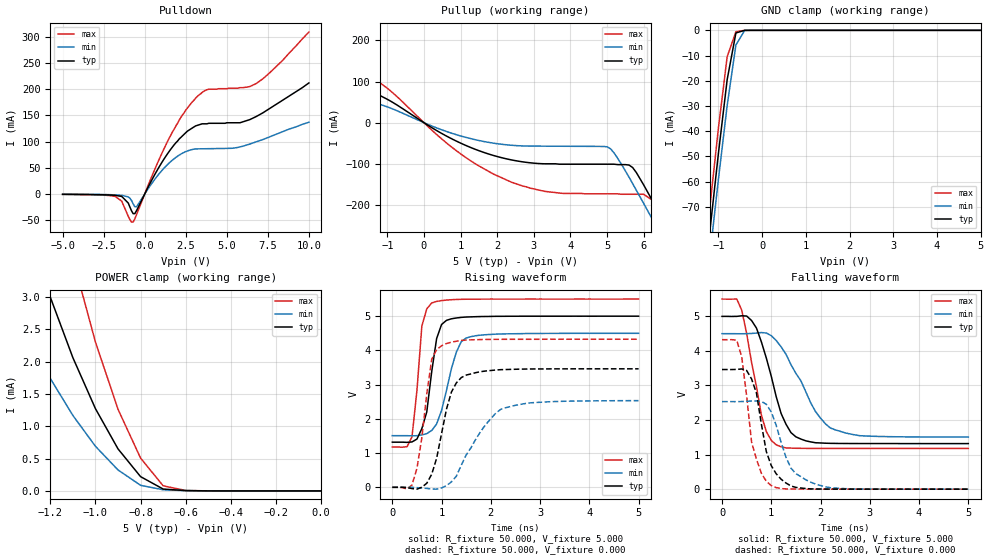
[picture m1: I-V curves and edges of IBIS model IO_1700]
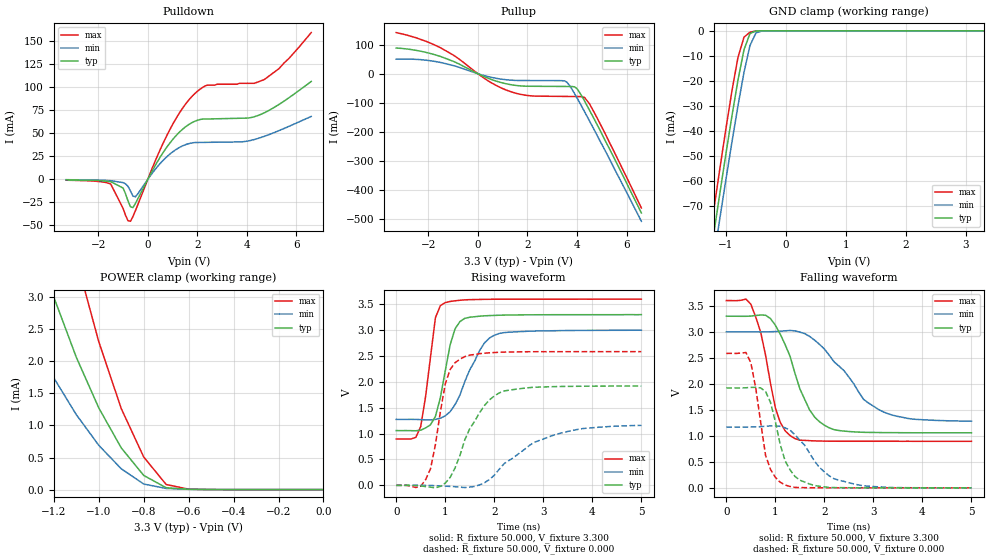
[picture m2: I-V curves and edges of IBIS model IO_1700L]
| / 7\'7   Xilinx XC1700 I/O Buffer IBIS File
| \ \   Xilinx Inc.
| / /   2100 Logic Drive
| \_\/.\   San Jose,   CA 95124
[IBIS ver]   2.1
[File name]   xc1700.ibs
[File Rev]   1.0
[Date]   July 26, 1999
[Source]   Spice netlist
[Notes]   - Best/worse process data included in the model
   - Created by Joey Jia x4437
[Disclaimer] The data in this model is derived from SPICE simulations
   using modeling information extracted from the target pro-
   cess. While a great deal of care has been take to provide
   information that is accurate, this model is considered
   preliminary as it has not been verified by actual silicon
   measurement. Treat the data in this model as preliminary
   until actual silicon verification is performed.
[Copyright]   Xilinx Inc. All right reserved
|   Component XC1701_PC20
[Component]   XC1701_PC20
[Manufacturer]   Xilinx Inc.
[Package]
| variable   typ   min   max
R_pkg   53.00m   49.000m   57.00m
L_pkg   3.125nH   2.880nH   3.370nH
C_pkg   0.650pF   0.630pF   0.670pF
[Pin]  signal_name   model_name   R_pin   L_pin   C_pin
io   datap   IO_1700   NA   NA   NA
| End [Component] XC1701_PC20
|   Component XC1701_PD8
[Component]   XC1701_PD8
[Manufacturer]   Xilinx Inc.
[Package]
| variable   typ   min   max
R_pkg   89.00m   80.000m   98.00m
L_pkg   5.840nH   4.160nH   7.520nH
C_pkg   0.935pF   0.720pF   1.150pF
[Pin]  signal_name   model_name   R_pin   L_pin   C_pin
io   datap   IO_1700   NA   NA   NA
| End [Component] XC1701_PD8
|   Component XC1701_SO20
[Component]   XC1701_SO20
[Manufacturer]   Xilinx Inc.
[Package]
| variable   typ   min   max
R_pkg   51.50m   44.000m   59.00m
L_pkg   3.155nH   1.960nH   4.350nH
C_pkg   0.585pF   0.350pF   0.820pF
[Pin]  signal_name   model_name   R_pin   L_pin   C_pin
io   datap   IO_1700   NA   NA   NA
| End [Component] XC1701_SO20
|   Component XC1701L_PC20
[Component]   XC1701L_PC20
[Manufacturer]   Xilinx Inc.
[Package]
| variable   typ   min   max
R_pkg   53.00m   49.000m   57.00m
L_pkg   3.125nH   2.880nH   3.370nH
C_pkg   0.650pF   0.630pF   0.670pF
[Pin]  signal_name   model_name   R_pin   L_pin   C_pin
io   datap   IO_1700L   NA   NA   NA
| End [Component] XC1701L_PC20
|   Component XC1701L_PD8
[Component]   XC1701L_PD8
[Manufacturer]   Xilinx Inc.
[Package]
| variable   typ   min   max
R_pkg   89.00m   80.000m   98.00m
L_pkg   5.840nH   4.160nH   7.520nH
C_pkg   0.935pF   0.720pF   1.150pF
[Pin]  signal_name   model_name   R_pin   L_pin   C_pin
io   datap   IO_1700L   NA   NA   NA
| End [Component] XC1701L_PD8
|   Component XC1701L_SO20
[Component]   XC1701L_SO20
[Manufacturer]   Xilinx Inc.
[Package]
| variable   typ   min   max
R_pkg   51.50m   44.000m   59.00m
L_pkg   3.155nH   1.960nH   4.350nH
C_pkg   0.585pF   0.350pF   0.820pF
[Pin]  signal_name   model_name   R_pin   L_pin   C_pin
io   datap   IO_1700L   NA   NA   NA
| End [Component] XC1701L_SO20
|   Component XC1702_PC44
[Component]   XC1702_PC44
[Manufacturer]   Xilinx Inc.
[Package]
| variable   typ   min   max
R_pkg   67.50m   66.000m   69.00m
L_pkg   3.905nH   3.550nH   4.260nH
C_pkg   0.895pF   0.790pF   1.000pF
[Pin]  signal_name   model_name   R_pin   L_pin   C_pin
io   datap   IO_1700L   NA   NA   NA
| End [Component] XC1702_PC44
|   Component XC1702_VQ44
[Component]   XC1702_VQ44
[Manufacturer]   Xilinx Inc.
[Package]
| variable   typ   min   max
R_pkg   54.15m   51.300m   57.00m
L_pkg   2.157nH   1.995nH   2.309nH
C_pkg   0.261pF   0.247pF   0.276pF
[Pin]  signal_name   model_name   R_pin   L_pin   C_pin
io   datap   IO_1700L   NA   NA   NA
| End [Component] XC1702_VQ44
|   Component XC1704_PC44
[Component]   XC1704_PC44
[Manufacturer]   Xilinx Inc.
[Package]
| variable   typ   min   max
R_pkg   67.50m   66.000m   69.00m
L_pkg   3.905nH   3.550nH   4.260nH
C_pkg   0.895pF   0.790pF   1.000pF
[Pin]  signal_name   model_name   R_pin   L_pin   C_pin
io   datap   IO_1700L   NA   NA   NA
| End [Component] XC1704_PC44
|   Component XC1704_VQ44
[Component]   XC1704_VQ44
[Manufacturer]   Xilinx Inc.
[Package]
| variable   typ   min   max
R_pkg   54.15m   51.300m   57.00m
L_pkg   2.157nH   1.995nH   2.309nH
C_pkg   0.261pF   0.247pF   0.276pF
[Pin]  signal_name   model_name   R_pin   L_pin   C_pin
io   datap   IO_1700L   NA   NA   NA
| End [Component] XC1704_VQ44
|   Component XC17512_PC20
[Component]   XC17512_PC20
[Manufacturer]   Xilinx Inc.
[Package]
| variable   typ   min   max
R_pkg   53.00m   49.000m   57.00m
L_pkg   3.125nH   2.880nH   3.370nH
C_pkg   0.650pF   0.630pF   0.670pF
[Pin]  signal_name   model_name   R_pin   L_pin   C_pin
io   datap   IO_1700   NA   NA   NA
| End [Component] XC17512_PC20
|   Component XC17512_PD8
[Component]   XC17512_PD8
[Manufacturer]   Xilinx Inc.
[Package]
| variable   typ   min   max
R_pkg   89.00m   80.000m   98.00m
L_pkg   5.840nH   4.160nH   7.520nH
C_pkg   0.935pF   0.720pF   1.150pF
[Pin]  signal_name   model_name   R_pin   L_pin   C_pin
io   datap   IO_1700   NA   NA   NA
| End [Component] XC17512_PD8
|   Component XC17512_SO20
[Component]   XC17512_SO20
[Manufacturer]   Xilinx Inc.
[Package]
| variable   typ   min   max
R_pkg   51.50m   44.000m   59.00m
L_pkg   3.155nH   1.960nH   4.350nH
C_pkg   0.585pF   0.350pF   0.820pF
[Pin]  signal_name   model_name   R_pin   L_pin   C_pin
io   datap   IO_1700   NA   NA   NA
| End [Component] XC17512_SO20
|   Component XC17512L_PC20
[Component]   XC17512L_PC20
[Manufacturer]   Xilinx Inc.
[Package]
| variable   typ   min   max
R_pkg   53.00m   49.000m   57.00m
L_pkg   3.125nH   2.880nH   3.370nH
C_pkg   0.650pF   0.630pF   0.670pF
[Pin]  signal_name   model_name   R_pin   L_pin   C_pin
io   datap   IO_1700L   NA   NA   NA
| End [Component] XC17512L_PC20
|   Component XC17512L_PD8
[Component]   XC17512L_PD8
[Manufacturer]   Xilinx Inc.
[Package]
| variable   typ   min   max
R_pkg   89.00m   80.000m   98.00m
L_pkg   5.840nH   4.160nH   7.520nH
C_pkg   0.935pF   0.720pF   1.150pF
[Pin]  signal_name   model_name   R_pin   L_pin   C_pin
io   datap   IO_1700L   NA   NA   NA
| End [Component] XC17512L_PD8
|   Component XC17512L_SO20
[Component]   XC17512L_SO20
[Manufacturer]   Xilinx Inc.
[Package]
| variable   typ   min   max
R_pkg   51.50m   44.000m   59.00m
L_pkg   3.155nH   1.960nH   4.350nH
C_pkg   0.585pF   0.350pF   0.820pF
[Pin]  signal_name   model_name   R_pin   L_pin   C_pin
io   datap   IO_1700L   NA   NA   NA
| End [Component] XC17512L_SO20
| Models and submodels in the file (2): IO_1700 (I/O), IO_1700L (I/O)
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|   Model IO_1700
[Model]   IO_1700
Model_type   I/O
Polarity   Non-Inverting
Enable   Active-High
Vinl =   0.800V
Vinh =   2.000V
Vmeas =   2.500V
Cref =  50.000pF
Rref =   1.000M
Vref =  0.000V
C_comp   2.750pF   2.250pF   3.250pF
[Temperature Range]   50.000   100.000   0.000
[Voltage Range]   5.000V   4.500V   5.500V
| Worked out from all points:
|   slope of the pulldown table from 0 to 0.75 V, typ, clamps not added: 16.8 ohm
|   slope of the pullup table from 0 to 0.75 V, typ, clamps not added: 19.3 ohm
|   GND clamp passes 1 mA (typ) near -0.59 V on its own axis
|   POWER clamp passes 1 mA (typ) near -0.96 V on its own axis
|   rising waveform, R_fixture 50.000, V_fixture 5.000: 20-80 % time 222ps typ, 325ps min, 154ps max; typ from 1.32 V to 5 V
|   rising waveform, R_fixture 50.000, V_fixture 0.000: 20-80 % time 331ps typ, 657ps min, 237ps max; typ from 0 V to 3.46 V
|   falling waveform, R_fixture 50.000, V_fixture 5.000: 20-80 % time 444ps typ, 672ps min, 339ps max; typ from 5 V to 1.32 V
|   falling waveform, R_fixture 50.000, V_fixture 0.000: 20-80 % time 296ps typ, 409ps min, 267ps max; typ from 3.46 V to 0 V
[Pulldown]
| voltage   I(typ)   I(min)   I(max)
-5V       -500uA     -400uA     -700uA
-1.8V     -2.5mA     -1.6mA     -4.5mA
-1.4V     -4.5mA     -2.4mA     -13.5mA
-1V       -17.19mA   -5.5mA     -42.5mA
-700mV    -37.46mA   -18.93mA   -53.28mA
-500mV    -31.8mA    -24.06mA   -39.58mA
1.4V      77.3mA     56.57mA    101mA
3.1V      130mA      86.12mA    183mA
3.9V      135mA      86.54mA    200mA
5.8V      136mA      89.89mA    203mA
6.8V      148mA      99.73mA    211mA
10V       212mA      137mA      309mA
[Pullup]
| voltage   I(typ)   I(min)   I(max)
-5V       138mA      75.48mA    233mA
-3.8V     136mA      79.24mA    211mA
-2.2V     104mA      68.39mA    154mA
-1V       56.81mA    38.43mA    83.6mA
1V        -49.62mA   -32.24mA   -75.63mA
2.4V      -90.7mA    -55.01mA   -145mA
3.3V      -100mA     -57.13mA   -167mA
5V        -101mA     -58.64mA   -173mA
5.7V      -109mA     -148mA     -174mA
6.4V      -215mA     -261mA     -198mA
6.8V      -281mA     -327mA     -262mA
10V       -833mA     -863mA     -828mA
[GND_clamp]
| voltage   I(typ)   I(min)   I(max)
-5V       -728mA     -719mA     -739mA
-1.4V     -113mA     -121mA     -104mA
-1.2V     -80.19mA   -89.89mA   -70.7mA
-1V       -48.75mA   -59.03mA   -38.71mA
-800mV    -19.55mA   -29.76mA   -10.47mA
-600mV    -1.037mA   -5.805mA   -545uA
-400mV    -3.699uA   -72.4uA    -2.038uA
5V        350pA      999nA      143pA
[POWER_clamp]
| voltage   I(typ)   I(min)   I(max)
-5V       71.66mA    42.52mA    116mA
-1.4V     5.246mA    3.126mA    8.7mA
-1.3V     4.067mA    2.398mA    6.818mA
-1.2V     3.001mA    1.742mA    5.11mA
-1.1V     2.064mA    1.169mA    3.598mA
-1V       1.274mA    691uA      2.306mA
-900mV    651uA      325uA      1.264mA
-800mV    221uA      87.03uA    508uA
-700mV    28.94uA    18.03uA    79.19uA
-600mV    5.041uA    4.416uA    6.917uA
0V        350pA      2.497nA    186pA
[Ramp]
| variable   typ   min   max
dV/dt_r   2.077/0.321n   1.520/0.637n   2.596/0.184n
dV/dt_f   2.209/0.440n   1.795/0.668n   2.593/0.308n
R_load = 50.000
[Rising Waveform]
R_fixture = 50.000
V_fixture = 5.000
V_fixture_min = 4.500
V_fixture_max = 5.500
L_fixture = 0.000H
C_fixture = 0.000F
| time   V(typ)   V(min)   V(max)
0s        1.319V     1.509V     1.178V
400ps     1.326V     1.504V     1.474V
600ps     1.716V     1.53V      4.712V
700ps     2.203V     1.569V     5.214V
800ps     3.381V     1.66V      5.387V
900ps     4.347V     1.851V     5.431V
1ns       4.757V     2.245V     5.455V
1.3ns     4.947V     3.95V      5.488V
1.5ns     4.975V     4.362V     5.495V
5ns       5V         4.499V     5.5V
[Rising Waveform]
R_fixture = 50.000
V_fixture = 0.000
V_fixture_min = 0.000
V_fixture_max = 0.000
L_fixture = 0.000H
C_fixture = 0.000F
| time   V(typ)   V(min)   V(max)
0s        0V         0V         0V
400ps     -36.91mV   -1.493mV   68.88mV
600ps     2.791mV    -20.69mV   1.452V
800ps     381mV      -52.4mV    3.743V
1ns       1.57V      -19.69mV   4.136V
1.2ns     2.782V     158mV      4.242V
1.3ns     3.05V      324mV      4.268V
1.8ns     3.38V      1.644V     4.317V
2.2ns     3.437V     2.277V     4.324V
5ns       3.462V     2.533V     4.326V
[Falling Waveform]
R_fixture = 50.000
V_fixture = 5.000
V_fixture_min = 4.500
V_fixture_max = 5.500
L_fixture = 0.000H
C_fixture = 0.000F
| time   V(typ)   V(min)   V(max)
0s        5V         4.5V       5.5V
300ps     5V         4.498V     5.501V
400ps     5.017V     4.497V     5.182V
600ps     4.881V     4.506V     3.67V
800ps     4.259V     4.532V     2.14V
1.1ns     2.678V     4.303V     1.284V
1.4ns     1.636V     3.604V     1.189V
1.9ns     1.343V     2.242V     1.179V
2.2ns     1.326V     1.77V      1.179V
5ns       1.319V     1.509V     1.178V
[Falling Waveform]
R_fixture = 50.000
V_fixture = 0.000
V_fixture_min = 0.000
V_fixture_max = 0.000
L_fixture = 0.000H
C_fixture = 0.000F
| time   V(typ)   V(min)   V(max)
0s        3.462V     2.534V     4.326V
300ps     3.466V     2.533V     4.308V
400ps     3.478V     2.535V     3.832V
600ps     3.19V      2.551V     1.364V
700ps     2.777V     2.552V     865mV
800ps     1.875V     2.538V     458mV
1ns       681mV      2.234V     103mV
1.4ns     92.11mV    608mV      4.998mV
1.8ns     7.997mV    202mV      1.287mV
5ns       186uV      382uV      121uV
|   Model IO_1700L
[Model]   IO_1700L
Model_type   I/O
Polarity   Non-Inverting
Enable   Active-High
Vinl =   0.800V
Vinh =   2.000V
Vmeas =   1.650V
Cref =  50.000pF
Rref =   1.000M
Vref =  0.000V
C_comp   2.750pF   2.250pF   3.250pF
[Temperature Range]   50.000   100.000   0.000
[Voltage Range]   3.300V   3.000V   3.600V
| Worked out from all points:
|   slope of the pulldown table from 0 to 0.495 V, typ, clamps not added: 20.8 ohm
|   slope of the pullup table from 0 to 0.495 V, typ, clamps not added: 27 ohm
|   GND clamp passes 1 mA (typ) near -0.60 V on its own axis
|   POWER clamp passes 1 mA (typ) near -0.96 V on its own axis
|   rising waveform, R_fixture 50.000, V_fixture 3.300: 20-80 % time 295ps typ, 502ps min, 225ps max; typ from 1.06 V to 3.3 V
|   rising waveform, R_fixture 50.000, V_fixture 0.000: 20-80 % time 575ps typ, 1.05ns min, 297ps max; typ from 0 V to 1.92 V
|   falling waveform, R_fixture 50.000, V_fixture 3.300: 20-80 % time 543ps typ, 897ps min, 359ps max; typ from 3.3 V to 1.06 V
|   falling waveform, R_fixture 50.000, V_fixture 0.000: 20-80 % time 348ps typ, 613ps min, 271ps max; typ from 1.92 V to 0 V
[Pulldown]
| voltage   I(typ)   I(min)   I(max)
-3.3V     -600uA     -400uA     -1mA
-1.5V     -2.5mA     -1.5mA     -5mA
-1V       -9.44mA    -3.56mA    -31.42mA
-800mV    -23.41mA   -7.59mA    -44.81mA
-700mV    -29.72mA   -12.65mA   -45.51mA
-500mV    -26.19mA   -18.96mA   -34.02mA
700mV     32.2mA     22.71mA    43.69mA
1.8V      61.63mA    39.51mA    90.28mA
2.4V      65.36mA    40.06mA    102mA
4.7V      71.97mA    46.5mA     108mA
5.3V      81.16mA    52.79mA    120mA
6.6V      106mA      68.14mA    159mA
[Pullup]
| voltage   I(typ)   I(min)   I(max)
-3.3V     88.66mA    50.5mA     142mA
-1.5V     59.21mA    38.72mA    89.11mA
-900mV    39.17mA    25.89mA    59mA
400mV     -15.21mA   -9.642mA   -23.79mA
1.2V      -35.64mA   -21.22mA   -58.08mA
2.1V      -43.2mA    -23.48mA   -76.02mA
3.6V      -43.97mA   -29.75mA   -78.34mA
4V        -51.68mA   -83.1mA    -78.68mA
4.3V      -93.08mA   -130mA     -81.45mA
4.5V      -125mA     -162mA     -103mA
5.1V      -224mA     -259mA     -200mA
6.6V      -480mA     -509mA     -463mA
[GND_clamp]
| voltage   I(typ)   I(min)   I(max)
-3.3V     -434mA     -434mA     -435mA
-1.3V     -96.3mA    -106mA     -87.19mA
-1.2V     -80.19mA   -89.89mA   -70.7mA
-1.1V     -64.31mA   -74.33mA   -54.49mA
-1V       -48.75mA   -59.03mA   -38.71mA
-900mV    -33.69mA   -44.1mA    -23.71mA
-800mV    -19.54mA   -29.76mA   -10.47mA
-700mV    -7.504mA   -16.51mA   -2.514mA
-600mV    -1.037mA   -5.805mA   -545uA
-500mV    -70.45uA   -808uA     -33.21uA
-400mV    -3.698uA   -72.41uA   -2.036uA
3.3V      204pA      39.97nA    67.46pA
[POWER_clamp]
| voltage   I(typ)   I(min)   I(max)
-3.3V     38.24mA    23.14mA    61.44mA
-1.4V     5.246mA    3.126mA    8.7mA
-1.3V     4.067mA    2.398mA    6.818mA
-1.2V     3.001mA    1.742mA    5.11mA
-1.1V     2.064mA    1.169mA    3.598mA
-1V       1.274mA    691uA      2.306mA
-900mV    651uA      325uA      1.264mA
-800mV    221uA      87.03uA    508uA
-700mV    28.94uA    18.03uA    79.19uA
-600mV    5.041uA    4.415uA    6.917uA
0V        204pA      1.705nA    79.84pA
[Ramp]
| variable   typ   min   max
dV/dt_r   1.152/0.573n   0.695/1.045n   1.551/0.280n
dV/dt_f   1.345/0.540n   1.031/0.916n   1.623/0.342n
R_load = 50.000
[Rising Waveform]
R_fixture = 50.000
V_fixture = 3.300
V_fixture_min = 3.000
V_fixture_max = 3.600
L_fixture = 0.000H
C_fixture = 0.000F
| time   V(typ)   V(min)   V(max)
0s        1.059V     1.275V     895mV
400ps     1.055V     1.275V     928mV
500ps     1.067V     1.271V     1.136V
800ps     1.334V     1.274V     3.242V
1ns       2.212V     1.343V     3.533V
1.1ns     2.716V     1.424V     3.555V
1.3ns     3.166V     1.746V     3.578V
1.7ns     3.27V      2.604V     3.594V
2ns       3.285V     2.902V     3.598V
5ns       3.3V       2.999V     3.6V
[Rising Waveform]
R_fixture = 50.000
V_fixture = 0.000
V_fixture_min = 0.000
V_fixture_max = 0.000
L_fixture = 0.000H
C_fixture = 0.000F
| time   V(typ)   V(min)   V(max)
0s        0V         0V         0V
600ps     -23.15mV   -251uV     110mV
700ps     -34.32mV   -2.234mV   321mV
1ns       42.35mV    -15.78mV   1.959V
1.3ns     578mV      -35.37mV   2.439V
1.5ns     1.096V     -33.89mV   2.517V
1.8ns     1.543V     50.44mV    2.554V
2.2ns     1.824V     419mV      2.576V
3.3ns     1.91V      995mV      2.584V
5ns       1.92V      1.159V     2.585V
[Falling Waveform]
R_fixture = 50.000
V_fixture = 3.300
V_fixture_min = 3.000
V_fixture_max = 3.600
L_fixture = 0.000H
C_fixture = 0.000F
| time   V(typ)   V(min)   V(max)
0s        3.3V       3V         3.6V
500ps     3.302V     2.998V     3.53V
700ps     3.323V     2.997V     2.995V
1ns       3.126V     3.005V     1.538V
1.2ns     2.752V     3.019V     1.096V
1.4ns     2.201V     3.018V     947mV
1.7ns     1.495V     2.91V      907mV
2.2ns     1.118V     2.42V      897mV
3.2ns     1.062V     1.461V     896mV
5ns       1.059V     1.282V     895mV
[Falling Waveform]
R_fixture = 50.000
V_fixture = 0.000
V_fixture_min = 0.000
V_fixture_max = 0.000
L_fixture = 0.000H
C_fixture = 0.000F
| time   V(typ)   V(min)   V(max)
0s        1.921V     1.169V     2.585V
400ps     1.924V     1.168V     2.602V
500ps     1.931V     1.17V      2.405V
600ps     1.933V     1.173V     1.917V
800ps     1.853V     1.184V     626mV
1ns       1.273V     1.193V     201mV
1.2ns     516mV      1.154V     54.62mV
1.5ns     147mV      916mV      5.838mV
2.2ns     5.607mV    174mV      571uV
5ns       270uV      455uV      69.19uV
